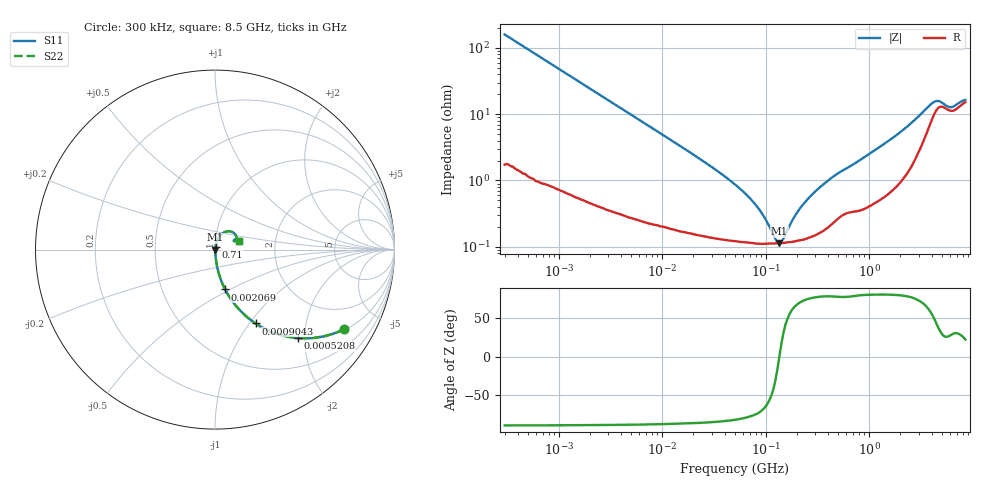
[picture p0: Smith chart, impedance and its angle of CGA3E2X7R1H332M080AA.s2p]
! S-parameter Generated by TDK Corporation
! Copyright(C) 2015 TDK Corporation.
! All Rights Reserved.
! TDK P/N: CGA3E2X7R1H332M080AA (Multilayer Ceramic Chip Capacitors)
! Property: C=3.3nF
! Size(LxWxT): 1.6x0.8x0.8mm, 0.063x0.031x0.031inches
! Model Type: s2p (Touchstone File Format Version 1.0)
! Frequency: DC=Yes Start=0.3MHz Stop=8500MHz 225points Log-sweep
! Note:
! Model Generated on Jun. 23, 2015
! Hash(MD5):
! Port Assignments:
!  1 ---| |--- 2
! Applicable Conditions:
!  Temperature = 25 degC
!  DC Bias Voltage = 0 V
!  Small Signal Operation
! Terms and conditions regarding TDK Simulation Models
! (1)This simulation model is being provided solely for informational purposes. Please refer to the specifications of the products in terms of detailed characteristics of such products.
! (2)In no event shall TDK Corporation of any of its subsidiaries be liable for any loss or damage arising, directly or indirectly,
!  From any information contained in this simulation model, including, but not limited to loss or damages arising from any inaccuracies, omissions or errors in connection with such information.
! (3)Any and all copyrights on this simulation model are owned by TDK Corporation.
!  Duplication or redistribution of this simulation model without prior written permission from TDK Corporation is prohibited.
! (4)This simulation model is subject to any modification or change without any prior notice.
! (5)Neither TDK Corporation nor any of its subsidiaries shall make any warranty, express or implied,
!  Including but not limited to the correctness, implied warranties of merchantability and fitness for a particular purpose with respect to this simulation models.
! (6)The use of this simulation model shall be deemed to have consented to the terms and conditions hereof.
# MHz S MA R 50
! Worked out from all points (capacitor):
!   224 points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, 300 kHz to 8.5 GHz, reference 50 ohm
!   read as one part in series: C = 3.3 nF near 314.1 kHz
!   lowest |Z| = 113 mohm at 135.7 MHz (marker M1)
!   series resonance near 135.4 MHz, so ESL is about 420 pH
!   S11 on the Smith chart (normalised r, x): 300 kHz: 1.03, -3.20; 520.8 kHz: 1.02, -1.86; 904.3 kHz: 1.02, -1.07; 2.069 MHz: 1.01, -0.47; 710 MHz: 1.01, +0.03; 8.5 GHz: 1.30, +0.13
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0.3  0.8438 -31.8  0.5275 57.5  0.5275 57.5  0.8438 -31.8
0.5208429  0.6762 -46.8  0.7286 42.5  0.7286 42.5  0.6762 -46.8
0.9042579  0.47 -61.1  0.8759 28.0  0.8759 28.0  0.47 -61.1
1.72111  0.2715 -73.2  0.9576 15.8  0.9576 15.8  0.2715 -73.2
2.068572  0.229 -75.7  0.9691 13.2  0.9691 13.2  0.229 -75.7
4.122422  0.1182 -81.8  0.99 6.8  0.99 6.8  0.1182 -81.8
9.430415  0.0523 -84.8  0.9966 3.0  0.9966 3.0  0.0523 -84.8
51.67171  0.008457 -81.3  0.9988 0.5  0.9988 0.5  0.008457 -81.3
85.6787  0.003744 -72.6  0.9989 0.2  0.9989 0.2  0.003744 -72.6
123.7646  0.001317 -31.4  0.9989 0.0  0.9989 0.0  0.001317 -31.4
135.6836  0.001131 0.9  0.9989 -0.0  0.9989 -0.0  0.001131 0.9
148.7505  0.001335 31.6  0.9989 -0.0  0.9989 -0.0  0.001335 31.6
205.2186  0.003439 68.8  0.9988 -0.2  0.9988 -0.2  0.003439 68.8
283.1228  0.006211 76.3  0.9986 -0.3  0.9986 -0.3  0.006211 76.3
428.2171  0.01083 78.0  0.9978 -0.6  0.9978 -0.6  0.01083 78.0
710.042  0.01764 78.0  0.9965 -1.0  0.9965 -1.0  0.01764 78.0
1551.304  0.0398 78.6  0.9929 -2.3  0.9929 -2.3  0.0398 78.6
2819.992  0.08285 70.5  0.9755 -4.6  0.9755 -4.6  0.08285 70.5
4073.536  0.135 47.9  0.9151 -6.3  0.9151 -6.3  0.135 47.9
4675.929  0.1401 32.4  0.885 -4.9  0.885 -4.9  0.1401 32.4
6161.135  0.1145 25.2  0.8977 -3.1  0.8977 -3.1  0.1145 25.2
8500  0.1428 19.4  0.8666 -3.1  0.8666 -3.1  0.1428 19.4
